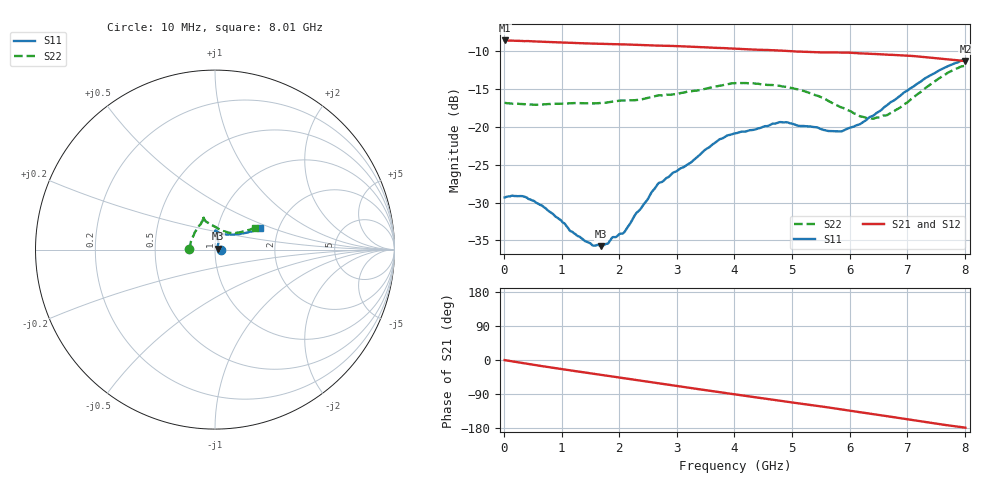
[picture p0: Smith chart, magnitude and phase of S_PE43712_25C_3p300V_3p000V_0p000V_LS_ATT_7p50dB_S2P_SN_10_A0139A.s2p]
! DEVICE ID: PE43712
! File Path: z:\PE43713\PE43713_CHAR_NOM_04292014\AMB\3p300\LS_ATT_7p50dB\PE43713_AMB_3p300V_3p000V_0p000V_LS_ATT_7p50dB_S2P_SN_10_A0139A.s2p
! Serial: 10
! Lot: A0139A
! Temp: 25C
! VDD: 3.300
! VSS: 0.000
! Control_Hi: 3.000
! Control_Lo: 0.000
! Attenuation Step: 7.50dB
! Port 1: RF1
! Port 2: RF2
! ThroughPath:1-2
! IDD: 0.0001474931
! ISS: -1.27e-007
#  Hz  S  RI  R  50
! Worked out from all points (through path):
!   801 points, 10 MHz to 8.01 GHz, reference 50 ohm
!   highest |S21| = -8.65 dB at 10 MHz (marker M1); lowest = -11.4 dB at 8.01 GHz (marker M2)
!   group delay of S21, straight-line fit = 61.3 ps
!   lowest |S11| = -35.8 dB at 1.68 GHz (marker M3), VSWR 1.03, Z = 51.6 + j0.546 ohm
!   |S11| at or under -10 dB: start of sweep to end of sweep
!   |S22| runs from -19.0 to -12.0 dB; largest |S21 - S12| = 0.0012
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1e7  0.0341 8.16e-05  0.3696 -0.00197  0.3696 -0.00191  -0.1436 0.000879
3e8  0.0346 -0.00442  0.3638 -0.0485  0.3637 -0.0485  -0.1401 0.0142
5e8  0.032 -0.00612  0.356 -0.0785  0.3561 -0.0785  -0.1378 0.0226
6.9e8  0.0288 -0.00631  0.3466 -0.1052  0.3466 -0.1052  -0.1363 0.0322
1.35e9  0.0183 -0.00139  0.3011 -0.1866  0.3012 -0.1867  -0.1284 0.0618
1.55e9  0.0163 0.00223  0.2842 -0.2083  0.2842 -0.2083  -0.1226 0.0721
1.68e9  0.0154 0.00529  0.2726 -0.2215  0.2726 -0.2215  -0.1198 0.0784
2.09e9  0.0138 0.0148  0.2318 -0.2594  0.2319 -0.2593  -0.1111 0.0988
2.68e9  0.0189 0.0378  0.1642 -0.2997  0.1641 -0.2997  -0.0863 0.1355
3.24e9  0.0148 0.0559  0.0936 -0.3228  0.0936 -0.3229  -0.0737 0.1539
3.72e9  0.0125 0.0803  0.0326 -0.3284  0.0323 -0.3283  -0.0676 0.1725
4.01e9  0.00856 0.0899  -0.00409 -0.3265  -0.00414 -0.3264  -0.0696 0.1805
4.79e9  0.00263 0.1071  -0.0954 -0.3022  -0.0955 -0.3025  -0.0633 0.1744
5.35e9  0.0137 0.0987  -0.1521 -0.2704  -0.152 -0.2702  -0.0506 0.1566
5.63e9  0.0253 0.0901  -0.1775 -0.2521  -0.1775 -0.2522  -0.0312 0.1443
5.87e9  0.0376 0.0854  -0.2005 -0.2335  -0.2002 -0.2335  -0.0108 0.1331
6.18e9  0.0612 0.0838  -0.2248 -0.2045  -0.2244 -0.2047  0.0207 0.1151
6.34e9  0.0778 0.0848  -0.2357 -0.1891  -0.2352 -0.1891  0.038 0.1074
6.68e9  0.1132 0.085  -0.255 -0.1532  -0.2546 -0.1534  0.076 0.0941
7.35e9  0.1883 0.098  -0.2756 -0.0762  -0.2753 -0.0762  0.1534 0.1006
7.73e9  0.227 0.1099  -0.2748 -0.0341  -0.2747 -0.0343  0.1986 0.1138
8.01e9  0.2504 0.1224  -0.2702 -0.00669  -0.2699 -0.00717  0.2203 0.1214
